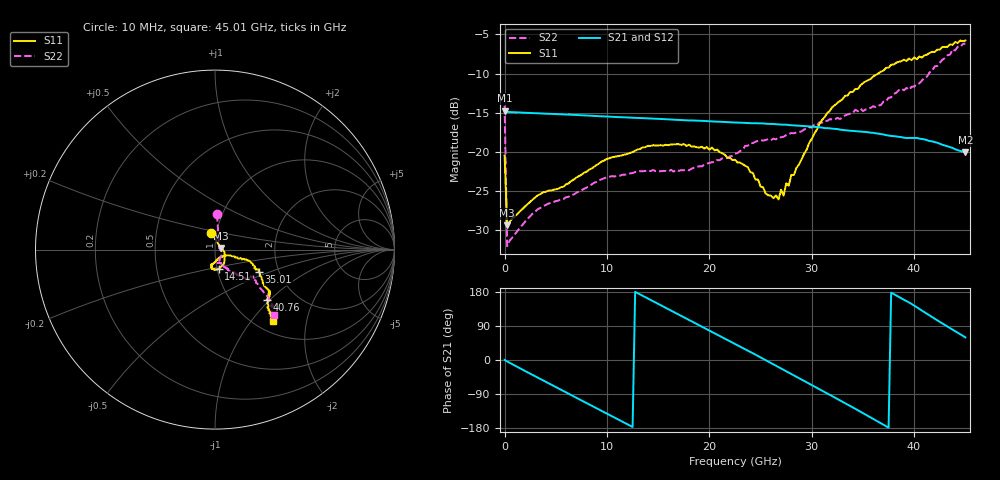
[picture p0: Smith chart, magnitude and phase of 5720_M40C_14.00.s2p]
! Device:  ADRF5720
! Description: 0.5dB LSB GaAs MMIC 6-bit Digital Attenuator
! Frequency:  0.000009 -  40 GHz
! Ports:
!	RF1	= Port 1
!	RF2	= Port 2
! Vdd:  3.3 Volt
! Vss:  -3.3 Volt
! Control:  0/3.3 Volt
! State:  14.00 dB attenuation
! Data:  The device was measured using G-S-G Probes on a matrix board.
!  Data was collected using an calibrated 4 port network analyzer.
!  The reference plane for this measurement is at the launchers.
! Note:  Analog Devices supplies this data as a sample of measured data
!  for this product.  Your particular data for this product may vary.
!  Data was taken at -40 degrees C.
!  Analog Devices reserves the right to change this data at anytime.
# GHZ S DB R 45.0
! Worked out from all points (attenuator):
!   181 points, 10 MHz to 45.01 GHz, reference 45 ohm
!   highest |S21| = -14.72 dB at 10 MHz (marker M1); lowest = -20.0 dB at 45.01 GHz (marker M2)
!   lowest |S11| = -29.3 dB at 260 MHz (marker M3), VSWR 1.07, Z = 48.1 + j0.835 ohm
!   |S11| at or under -10 dB: start of sweep to 36.5 GHz
!   |S22| runs from -32.0 to -6.2 dB; largest |S21 - S12| = 0.00069
!   S11 on the Smith chart (normalised r, x): 10 MHz: 0.94, +0.18; 14.51 GHz: 1.02, -0.22; 35.01 GHz: 1.58, -0.43; 40.76 GHz: 1.44, -0.95; 45.01 GHz: 1.19, -1.29
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0.01  -20.46 102.1  -14.72 0.2  -14.74 0.2  -14.11 86.8
0.26  -29.34 14.7  -14.90 -3.9  -14.92 -3.9  -32.00 18.0
3.26  -25.51 -12.8  -15.07 -46.8  -15.10 -46.8  -27.28 -27.5
7.76  -22.65 -43.4  -15.33 -110.1  -15.36 -110.2  -24.69 -61.5
11.26  -20.49 -61.5  -15.56 -159.2  -15.58 -159.2  -23.02 -74.2
14.51  -19.13 -78.8  -15.75 155.2  -15.77 155.1  -22.30 -79.3
15.26  -19.13 -82.3  -15.79 144.6  -15.81 144.5  -22.45 -79.0
19.01  -19.44 -97.0  -16.02 91.8  -16.04 91.7  -21.82 -69.1
22.76  -21.34 -104.2  -16.25 38.8  -16.28 38.7  -20.13 -62.9
23.76  -21.93 -99.0  -16.32 24.6  -16.34 24.5  -19.21 -61.9
25.51  -25.30 -75.7  -16.40 -0.6  -16.42 -0.7  -18.47 -58.4
26.76  -26.05 -50.7  -16.50 -18.6  -16.52 -18.8  -18.11 -57.0
27.01  -24.81 -46.1  -16.51 -22.1  -16.53 -22.3  -18.13 -58.5
27.26  -25.57 -42.8  -16.52 -25.8  -16.54 -25.9  -18.05 -56.6
27.51  -24.00 -36.9  -16.52 -29.4  -16.54 -29.6  -17.84 -57.8
27.76  -24.29 -33.2  -16.57 -33.2  -16.60 -33.3  -17.71 -56.0
30.26  -17.66 -18.7  -16.79 -69.8  -16.81 -69.9  -16.53 -55.8
32.01  -14.28 -18.4  -17.03 -95.6  -17.05 -95.7  -15.85 -52.0
35.01  -11.23 -27.1  -17.43 -139.9  -17.46 -140.1  -14.79 -48.2
37.76  -8.89 -37.0  -17.96 177.8  -17.98 177.7  -13.04 -44.9
40.76  -7.96 -44.0  -18.34 130.7  -18.37 130.5  -10.90 -37.1
45.01  -5.79 -51.0  -20.04 59.7  -20.07 59.5  -6.18 -48.0
